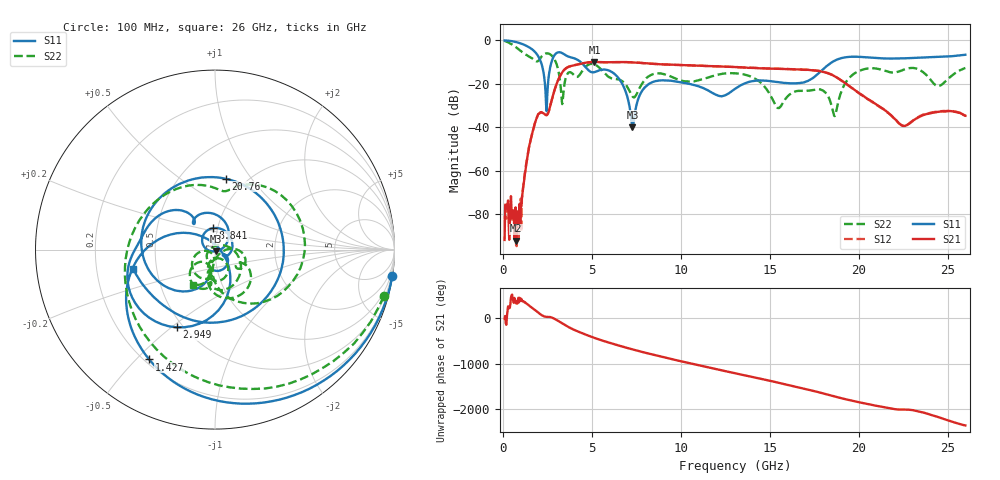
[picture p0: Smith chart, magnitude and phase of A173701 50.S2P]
!  2-Port S-parameters saved by WinCal
! VAR MeasName=S-Parameters (CALIBRATED_DATA) read from VNA (N5245A)
! VAR MeasDate=2017-6-7 10:31:45
! VAR NAME=A173701 50
! VAR FILENAME=A173701 50.S2P
! VAR DATE=2017-6-7 10:31:45
! VAR PHYS_PORTS=1,2
# Hz S DB R 50
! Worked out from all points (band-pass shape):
!   801 points, 100 MHz to 26 GHz, reference 50 ohm
!   highest |S21| = -9.90 dB at 5.151 GHz (marker M1); lowest = -92.1 dB at 747.5 MHz (marker M2)
!   |S21| within 3 dB of the highest: 3.536 GHz to 14.79 GHz (11.25 GHz wide, 123 % of centre)
!   lowest |S11| = -39.9 dB at 7.287 GHz (marker M3), VSWR 1.02, Z = 50.3 - j0.972 ohm
!   |S11| at or under -10 dB: 2.142 GHz to 2.733 GHz (590.5 MHz wide, 24.2 % of centre); 4.381 GHz to 18.5 GHz (14.12 GHz wide, 123 % of centre)
!   |S22| runs from -34.8 to -0.2 dB; largest |S21 - S12| = 0.0035
!   S11 on the Smith chart (normalised r, x): 100 MHz: 0, -13; 1.427 GHz: 0.22, -0.55; 2.949 GHz: 0.46, -0.52; 8.841 GHz: 0.95, +0.23; 20.76 GHz: 0.81, +0.76; 26 GHz: 0.37, -0.10
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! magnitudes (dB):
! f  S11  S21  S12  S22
! 100 MHz  0.0  -91.8  -81.0  -0.2
! 747.5 MHz  -0.8  -92.1  -94.4  -3.2
! 1.427 GHz  -2.9  -51.2  -51.1  -7.2
! 1.945 GHz  -6.7  -34.8  -34.7  -9.6
! 2.431 GHz  -29.4  -34.4  -34.4  -6.0
! 2.949 GHz  -6.3  -21.8  -21.7  -9.4
! 3.337 GHz  -5.8  -14.7  -14.7  -29.3
! 4.438 GHz  -10.4  -10.6  -10.6  -14.4
! 5.151 GHz  -14.6  -9.9  -9.9  -11.0
! 6.478 GHz  -17.1  -10.0  -10.0  -17.9
! 7.287 GHz  -39.9  -10.1  -10.1  -25.7
! 8.744 GHz  -18.5  -10.9  -10.9  -15.2
! 8.841 GHz  -18.4  -11.0  -11.0  -15.2
! 13.05 GHz  -22.3  -12.2  -12.3  -15.1
! 15.48 GHz  -19.2  -13.1  -13.1  -31.1
! 17.39 GHz  -17.5  -13.8  -13.7  -22.9
! 18.65 GHz  -9.3  -16.5  -16.4  -34.8
! 19.43 GHz  -7.6  -20.8  -20.8  -17.7
! 20.76 GHz  -8.0  -28.2  -28.3  -12.8
! 21.69 GHz  -8.3  -33.5  -33.6  -14.5
! 24.48 GHz  -7.6  -32.9  -32.7  -21.0
! 26 GHz  -6.6  -34.7  -34.6  -12.7
